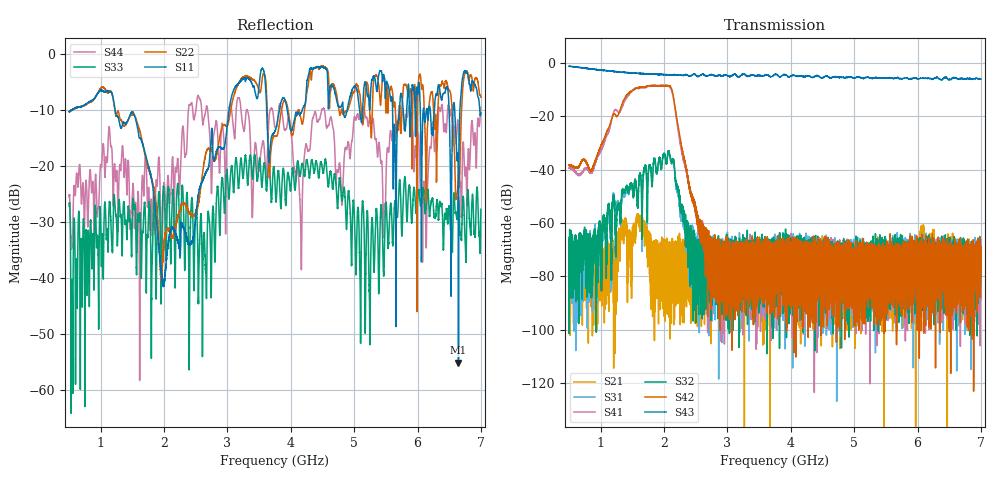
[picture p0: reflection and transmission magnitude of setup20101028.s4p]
!Agilent Technologies,E8364B,SG43040140,A.07.50.37
!Agilent E8364B: A.07.50.37
!Date: Thursday, October 28, 2010 13:34:13
!Correction: S11(Full 4 Port(1,2,3,4))
!S12(Full 4 Port(1,2,3,4))
!S13(Full 4 Port(1,2,3,4))
!S14(Full 4 Port(1,2,3,4))
!S21(Full 4 Port(1,2,3,4))
!S22(Full 4 Port(1,2,3,4))
!S23(Full 4 Port(1,2,3,4))
!S24(Full 4 Port(1,2,3,4))
!S31(Full 4 Port(1,2,3,4))
!S32(Full 4 Port(1,2,3,4))
!S33(Full 4 Port(1,2,3,4))
!S34(Full 4 Port(1,2,3,4))
!S41(Full 4 Port(1,2,3,4))
!S42(Full 4 Port(1,2,3,4))
!S43(Full 4 Port(1,2,3,4))
!S44(Full 4 Port(1,2,3,4))
!S4P File: Measurements: <S11,S12,S13,S14>,
!<S21,S22,S23,S24>,
!<S31,S32,S33,S34>,
!<S41,S42,S43,S44>:
# Hz S  dB  R 50
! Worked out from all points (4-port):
!   16000 points, 500 MHz to 7 GHz, reference 50 ohm
!   strongest paths, dB at 500 MHz, 2.125 GHz, 3.75 GHz, 5.375 GHz, 7 GHz:
!     S43: -1.3, -4.5, -4.4, -5.7, -6.2
!     S42: -38.4, -10.4, -76.3, -82.2, -75.5
!     S32: -66.7, -36.9, -70.9, -69.9, -73.2
!     S41: -39.5, -10.9, -77.4, -77.1, -88.4
!     S31: -69.9, -37.6, -77.2, -74.4, -79.0
!     S21: -71.1, -81.4, -79.0, -82.2, -69.2
!   lowest |S11| = -55.1 dB at 6.647 GHz (marker M1), VSWR 1.00, Z = 49.9 + j0.139 ohm
!   |S11| at or under -10 dB: 1.225 GHz to 3.026 GHz (1.802 GHz wide, 84.8 % of centre); 3.619 GHz to 3.819 GHz (200.4 MHz wide, 5.39 % of centre); 3.943 GHz to 4.182 GHz (238.5 MHz wide, 5.87 % of centre)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
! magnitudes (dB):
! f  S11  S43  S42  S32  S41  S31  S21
! 500 MHz  -10.4  -1.3  -38.4  -66.7  -39.5  -69.9  -71.1
! 939.2 MHz  -7.3  -2.6  -34.9  -75.6  -35.8  -74.8  -81.1
! 1.381 GHz  -12.4  -3.6  -13.2  -48.4  -14.2  -49.2  -61.5
! 2.102 GHz  -31.6  -4.5  -9.0  -35.8  -9.6  -36.6  -77.2
! 2.86 GHz  -16.7  -4.7  -69.4  -73.2  -82.3  -118.5  -82.9
! 6.647 GHz  -55.1  -6.2  -83.2  -80.9  -80.3  -82.3  -69.9
! 7 GHz  -10.5  -6.2  -75.5  -73.2  -88.4  -79.0  -69.2
